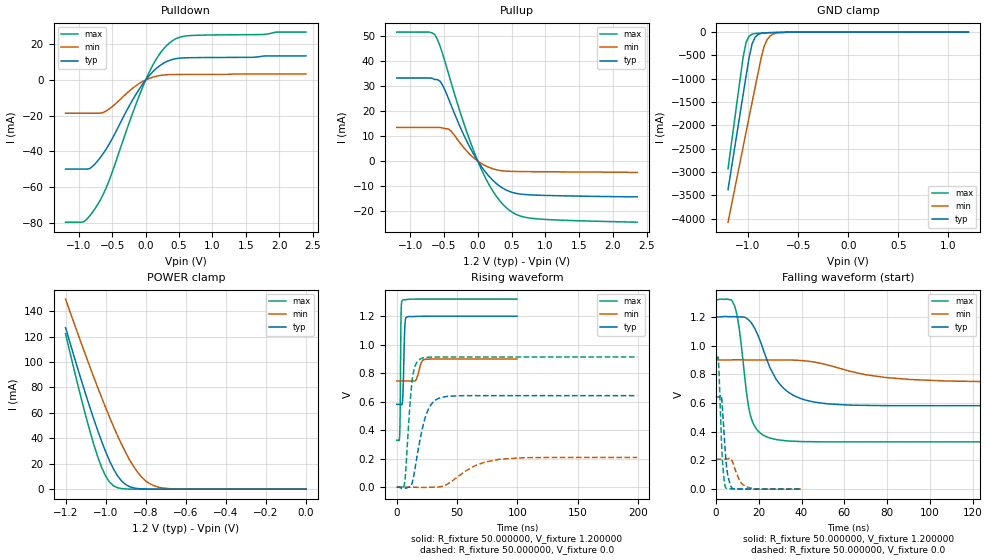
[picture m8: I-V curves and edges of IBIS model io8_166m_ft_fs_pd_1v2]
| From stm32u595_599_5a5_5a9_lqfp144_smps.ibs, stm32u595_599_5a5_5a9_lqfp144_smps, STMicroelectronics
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|   Model io8_166m_ft_fs_pd_1v2
[Model]  io8_166m_ft_fs_pd_1v2
Model_type I/O
Polarity   Non-Inverting
Enable   Active-Low
Vinl =   0.360000V
Vinh =   0.840000V
Vmeas =  0.600000V
Cref =   50.000000pF
Rref =   100.000000M
Vref =   0.0V
C_comp   3.151500pF   3.086800pF   3.197700pF
[Temperature Range]   25.000000   0.140000k   -40.000000
[Pullup Reference]   1.200000V   0.900000V   1.320000V
[Pulldown Reference]   0.0V   0.0V   0.0V
[POWER Clamp Reference]   1.200000V   0.900000V   1.320000V
[GND Clamp Reference]   0.0V   0.0V   0.0V
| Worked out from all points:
|   slope of the pulldown table from 0 to 0.18 V, typ, clamps not added: 25.4 ohm
|   slope of the pullup table from 0 to 0.18 V, typ, clamps not added: 27.8 ohm
|   GND clamp passes 1 mA (typ) near -0.51 V on its own axis
|   POWER clamp passes 1 mA (typ) near -0.86 V on its own axis
|   rising waveform, R_fixture 50.000000, V_fixture 1.200000: 20-80 % time 1.13ns typ, 3.03ns min, 570ps max; typ from 0.581 V to 1.2 V
|   rising waveform, R_fixture 50.000000, V_fixture 0.0: 20-80 % time 9.51ns typ, 24.6ns min, 4.59ns max; typ from 0 V to 0.642 V
|   falling waveform, R_fixture 50.000000, V_fixture 1.200000: 20-80 % time 12ns typ, 29.2ns min, 5.06ns max; typ from 1.2 V to 0.581 V
|   falling waveform, R_fixture 50.000000, V_fixture 0.0: 20-80 % time 1.94ns typ, 3.63ns min, 1.46ns max; typ from 0.642 V to 0 V
[Pulldown]
|Voltage   I(typ)   I(min)   I(max)
-1.2V     -49.86mA   -18.57mA   -79.56mA
-920mV    -49.86mA   -18.57mA   -79.19mA
-840mV    -49.6mA    -18.57mA   -76.08mA
-720mV    -45.32mA   -18.57mA   -69.74mA
-560mV    -36.71mA   -16.58mA   -57.44mA
-200mV    -11.43mA   -4.74mA    -19.03mA
0V        -10fA      -500fA     0A
160mV     6.477mA    2.075mA    11.78mA
360mV     10.99mA    2.99mA     20.81mA
480mV     12.07mA    3.054mA    23.53mA
640mV     12.43mA    3.075mA    24.76mA
2.4V      13.46mA    3.37mA     26.78mA
[Pullup]
|Voltage   I(typ)   I(min)   I(max)
-1.2V     33.36mA    13.53mA    51.76mA
-640mV    32.74mA    13.53mA    50.88mA
-560mV    32.1mA     13.53mA    46.17mA
-520mV    30.37mA    13.29mA    42.92mA
-400mV    22.74mA    12.14mA    31.92mA
-240mV    12.39mA    6.508mA    17.85mA
0V        0A         0A         0A
200mV     -7.072mA   -2.851mA   -11mA
440mV     -11.84mA   -4.03mA    -19.1mA
600mV     -13.07mA   -4.154mA   -21.71mA
840mV     -13.59mA   -4.223mA   -23.04mA
2.36V     -14.3mA    -4.5mA     -24.47mA
[GND_clamp]
|Voltage   I(typ)   I(min)   I(max)
-1.2V     -3.379A    -4.076A    -2.932A
-1.05V    -1.35A     -2.47A     -550.7mA
-1.02V    -947.8mA   -2.15A     -221.5mA
-990mV    -552.4mA   -1.829A    -88.45mA
-960mV    -255.3mA   -1.51A     -44.89mA
-930mV    -111.8mA   -1.191A    -30.7mA
-870mV    -28.37mA   -564.6mA   -21.36mA
-840mV    -18.66mA   -309.5mA   -18.51mA
-810mV    -14.08mA   -161.6mA   -15.94mA
-780mV    -11.38mA   -83.33mA   -13.55mA
-600mV    -3.02mA    -4.329mA   -3.104mA
1.2V      30.28uA    18.17uA    37.27uA
[POWER_clamp]
|Voltage   I(typ)   I(min)   I(max)
-1.2V     127mA      149.4mA    122.2mA
-1.12V    84.97mA    114mA      70.27mA
-1.06V    55.51mA    88.42mA    35.67mA
-1.02V    37.63mA    72.04mA    17.17mA
-1V       29.51mA    64.13mA    10.3mA
-960mV    15.69mA    48.99mA    2.571mA
-900mV    3.624mA    28.77mA    182.8uA
-840mV    490.7uA    13.24mA    11.35uA
-800mV    116.8uA    6.532mA    1.77uA
-740mV    13.2uA     1.724mA    109.1nA
-620mV    167.4nA    79.36uA    0A
0V        0A         17.87nA    0A
[Ramp]
| variable   typ   min   max
dV/dt_r  0.38524/9.50177n   0.12535/24.57552n   0.54788/4.57923n
dV/dt_f  0.37097/11.98615n   92.62200m/29.22329n 0.59419/5.05241n
R_load = 50.000000
[Rising Waveform]
R_fixture= 50.000000
V_fixture= 1.200000
V_fixture_min= 0.900000
V_fixture_max= 1.320000
|time   V(typ)   V(min)   V(max)
0s        581.2mV    745.1mV    329.2mV
2.402ns   581.3mV    745.1mV    367.4mV
2.803ns   581.3mV    745.1mV    517.5mV
3.203ns   580.8mV    745.1mV    965mV
3.604ns   579.6mV    745.1mV    1.238V
4.605ns   588.4mV    745.1mV    1.31V
6.607ns   1.113V     745.1mV    1.314V
8.008ns   1.192V     745.1mV    1.316V
22.82ns   1.199V     895.9mV    1.319V
99.7ns    1.2V       899.5mV    1.319V
[Rising Waveform]
R_fixture= 50.000000
V_fixture= 0.0
V_fixture_min= 0.0
V_fixture_max= 0.0
|time   V(typ)   V(min)   V(max)
0s        1.412uV    1.117uV    1.253uV
6.406ns   -3.83mV    408.9nV    25.35mV
10.81ns   773.8uV    3.324uV    563.1mV
12.81ns   32.74mV    37.78uV    752.4mV
15.22ns   135.2mV    -304.3uV   851.2mV
19.22ns   331.1mV    -1.29mV    898mV
26.83ns   557mV      -335.4uV   911.6mV
37.64ns   630.7mV    5.736mV    913mV
86.09ns   642mV      196.9mV    913.1mV
199.4ns   642.1mV    209.1mV    913.1mV
[Falling Waveform]
R_fixture= 50.000000
V_fixture= 1.200000
V_fixture_min= 0.900000
V_fixture_max= 1.320000
|time   V(typ)   V(min)   V(max)
0s        1.2V       899.5mV    1.319V
8.809ns   1.201V     900.6mV    1.271V
10.81ns   1.2V       900.6mV    1.122V
16.02ns   1.167V     899.8mV    518.7mV
19.22ns   1.085V     899.9mV    413.2mV
25.23ns   845.6mV    899.6mV    356mV
34.43ns   669.3mV    898.9mV    335.1mV
52.05ns   594.4mV    864.9mV    329.4mV
90.89ns   581.4mV    763.4mV    329.2mV
199.4ns   581.2mV    745.1mV    329.2mV
[Falling Waveform]
R_fixture= 50.000000
V_fixture= 0.0
V_fixture_min= 0.0
V_fixture_max= 0.0
|time   V(typ)   V(min)   V(max)
0s        642.1mV    209.1mV    913.1mV
1.201ns   641.9mV    209.1mV    876.4mV
2.563ns   643.3mV    209.1mV    331.8mV
3.443ns   465.4mV    209mV      119.3mV
4.484ns   233.7mV    208.7mV    11.27mV
5.445ns   103.2mV    210.7mV    4.185mV
7.528ns   6.267mV    197.5mV    2.078mV
11.53ns   1.162mV    48.84mV    723.9uV
15.46ns   648.9uV    10.45mV    298.1uV
39.88ns   1.412uV    1.117uV    1.253uV
